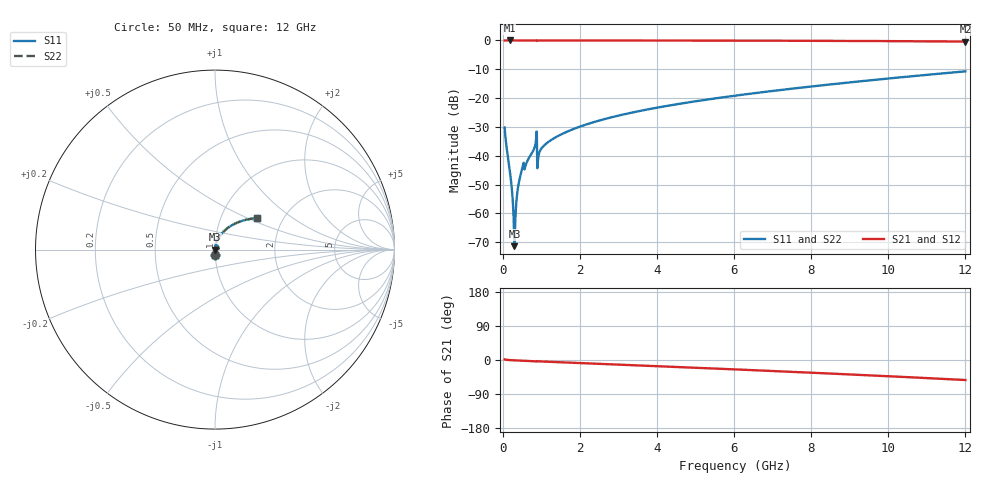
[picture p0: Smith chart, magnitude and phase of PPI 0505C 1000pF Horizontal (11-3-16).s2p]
# MHz S MA R 50
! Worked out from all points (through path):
!   1601 points, 50 MHz to 12 GHz, reference 50 ohm
!   highest |S21| = 0.00 dB at 177 MHz (marker M1); lowest = -0.4 dB at 12 GHz (marker M2)
!   group delay of S21, straight-line fit = 12.2 ps
!   lowest |S11| = -71.3 dB at 303.9 MHz (marker M3), VSWR 1.00, Z = 50 - j0.00751 ohm
!   |S11| at or under -10 dB: start of sweep to end of sweep
!   |S22| runs from -71.3 to -10.7 dB; largest |S21 - S12| = 0
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50  0.03093 -88.1  0.9994 1.6  0.9994 1.6  0.03093 -88.1
94.8125  0.01517 -88.7  0.9997 0.6  0.9997 0.6  0.01517 -88.7
176.9688  0.005999 -88.1  0.9997 -0.2  0.9997 -0.2  0.005999 -88.1
221.7812  0.003427 -86.5  0.9997 -0.5  0.9997 -0.5  0.003427 -86.5
251.6562  0.002072 -83.8  0.9997 -0.7  0.9997 -0.7  0.002072 -83.8
266.5938  0.001469 -80.9  0.9997 -0.7  0.9997 -0.7  0.001469 -80.9
303.9375  0.0002713 -16.1  0.9997 -0.9  0.9997 -0.9  0.0002713 -16.1
341.2812  0.001185 75.6  0.9997 -1.1  0.9997 -1.1  0.001185 75.6
408.5  0.003138 83.2  0.9997 -1.4  0.9997 -1.4  0.003138 83.2
490.6562  0.005459 84.2  0.9996 -1.8  0.9996 -1.8  0.005459 84.2
774.4688  0.01168 84.8  0.9994 -3.1  0.9994 -3.1  0.01168 84.8
826.75  0.01387 84.0  0.9992 -3.4  0.9992 -3.4  0.01387 84.0
953.7188  0.0116 83.5  0.9993 -3.6  0.9993 -3.6  0.0116 83.5
1035.875  0.01426 84.3  0.9994 -4.0  0.9994 -4.0  0.01426 84.3
1245  0.01856 83.8  0.9993 -4.9  0.9993 -4.9  0.01856 83.8
2044.156  0.03278 81.0  0.9989 -8.2  0.9989 -8.2  0.03278 81.0
2910.531  0.04812 77.6  0.9981 -11.7  0.9981 -11.7  0.04812 77.6
4038.312  0.06904 73.1  0.9967 -16.4  0.9967 -16.4  0.06904 73.1
6025  0.1102 64.8  0.9928 -24.8  0.9928 -24.8  0.1102 64.8
8019.156  0.1595 56.1  0.9858 -33.6  0.9858 -33.6  0.1595 56.1
10013.31  0.2193 46.9  0.974 -42.9  0.974 -42.9  0.2193 46.9
12000  0.2912 37.0  0.9547 -52.8  0.9547 -52.8  0.2912 37.0
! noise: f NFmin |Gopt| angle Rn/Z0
50  0.000288  0.8211  0.1894  0.0003375
1372  0.002507  0.5273  3.992  0.0009316
2701  0.004021  0.4503  7.489  0.001217
4031  0.005385  0.4079  10.71  0.001464
5360  0.006685  0.3815  13.68  0.0017
6682  0.007965  0.3655  16.4  0.001942
8012  0.009276  0.3573  18.97  0.002208
9341  0.01064  0.3558  21.4  0.00251
1.067e+04  0.01209  0.3601  23.79  0.002862
1.2e+04  0.01366  0.3697  26.18  0.003281
